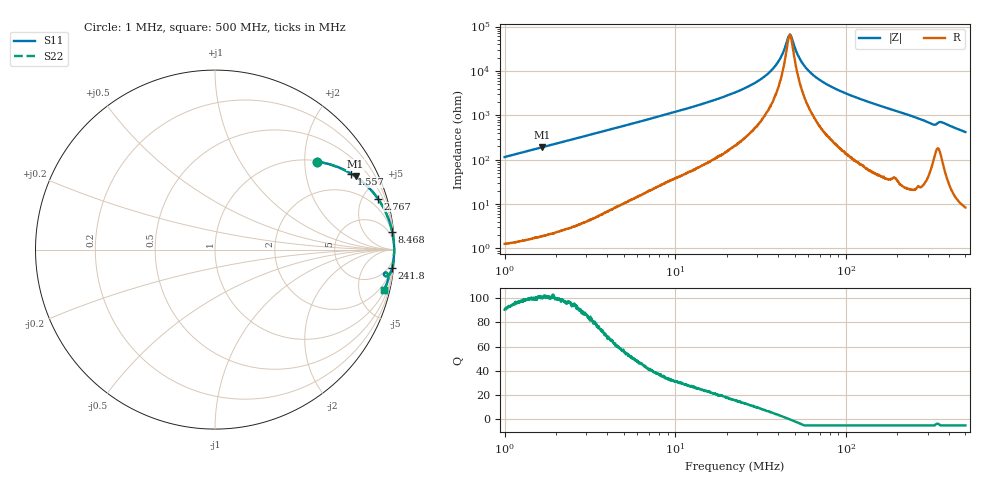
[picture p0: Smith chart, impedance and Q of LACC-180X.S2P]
!s-Parameter Generated by FASTRON Sdn. Bhd.
!FASTRON P/N : LACC-180X
!Keysight Technologies,E4991B,MY54100416,A.01.15
!Date: Wed Mar 18 09:32:54 2026
!Version  : Rev00 Wed Mar 18 09:32:54 2026
!Data & Calibration Information:
!PortZ  Port1:50+j0  Port2:50+j0
!When reading, reference impedance value at option line is always used.
!Remarks : This data is being provided solely for informational purposes.
!Freq	S11	S21	S12	S22
# Hz S dB R 50
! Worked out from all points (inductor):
!   1601 points, 1 MHz to 500 MHz, reference 50 ohm
!   read as one part in series: L = 18.3 uH near 1.032 MHz
!   highest Q = 101 at 1.663 MHz (marker M1), where L = 18.3 uH
!   self-resonance near 46.77 MHz
!   S11 on the Smith chart (normalised r, x): 1 MHz: 1.03, +2.30; 1.557 MHz: 1.04, +3.58; 2.767 MHz: 1.07, +6.37; 8.468 MHz: 2, +20; 241.8 MHz: 1, -19; 500 MHz: 1.17, -8.41
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1000000  -2.50 40.8  -3.70 -48.6  -3.70 -48.6  -2.50 40.8
1557047  -1.22 29.1  -6.27 -60.4  -6.27 -60.4  -1.22 29.1
1663329  -1.09 27.5  -6.72 -61.9  -6.72 -61.9  -1.09 27.5
2766663  -0.44 17.4  -10.50 -72.0  -10.50 -72.0  -0.44 17.4
2820919  -0.42 17.0  -10.66 -72.3  -10.66 -72.3  -0.42 17.0
7957584  -0.07 6.1  -19.50 -82.4  -19.50 -82.4  -0.07 6.1
8467807  -0.07 5.7  -20.06 -82.7  -20.06 -82.7  -0.07 5.7
2.236068e7  -0.02 1.7  -30.30 -84.6  -30.30 -84.6  -0.02 1.7
2.957595e7  -0.02 1.0  -34.86 -83.3  -34.86 -83.3  -0.02 1.0
3.619555e7  -0.02 0.6  -39.97 -79.6  -39.97 -79.6  -0.02 0.6
4.098591e7  -0.01 0.3  -45.43 -71.7  -45.43 -71.7  -0.01 0.3
4.569478e7  -0.01 0.1  -54.66 -30.5  -54.66 -30.5  -0.01 0.1
4.677219e7  -0.01 0.0  -56.21 -2.5  -56.21 -2.5  -0.01 0.0
4.806132e7  -0.01 -0.1  -54.83 31.6  -54.83 31.6  -0.01 -0.1
5.442207e7  -0.01 -0.3  -44.55 74.6  -44.55 74.6  -0.01 -0.3
6.307767e7  -0.01 -0.7  -38.65 81.9  -38.65 81.9  -0.01 -0.7
9.122775e7  -0.02 -1.6  -31.17 85.4  -31.17 85.4  -0.02 -1.6
1.77937e8  -0.04 -4.0  -23.04 84.5  -23.04 84.5  -0.04 -4.0
2.418399e8  -0.07 -5.9  -19.77 82.9  -19.77 82.9  -0.07 -5.9
3.211208e8  -0.28 -8.8  -16.23 73.8  -16.23 73.8  -0.28 -8.8
3.6362e8  -0.26 -7.9  -17.14 73.6  -17.14 73.6  -0.26 -7.9
5e8  -0.28 -13.3  -12.76 75.5  -12.76 75.5  -0.28 -13.3
